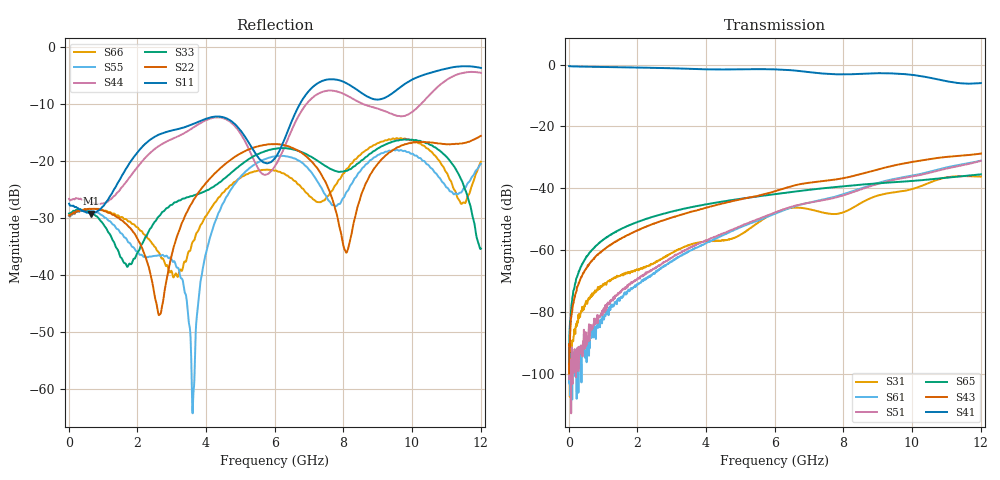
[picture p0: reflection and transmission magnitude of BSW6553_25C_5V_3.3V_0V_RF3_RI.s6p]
! Agilent Technologies	N5230C	MY49001333	A.09.33.09
!	Test time	=	2026-05-26
!	Product	=	BSW6553
!	Temp	=	25C
!	Logic	=	RF3
!	Port1	=	RFC
!	Port2	=	RF1
!	Port3	=	RF2
!	Port4	=	RF3
!	Port5	=	RF4
!	Port6	=	RF5
!S6P File: Measurements: <S11,S12,S13,S14,S15,S16>,
!<S21,S22,S23,S24,S25,S26>,
!<S31,S32,S33,S34,S35,S36>,
!<S41,S42,S43,S44,S45,S46>,
!<S51,S52,S53,S54,S55,S56>,
!<S61,S62,S63,S64,S65,S66>;
# HZ S RI R 50
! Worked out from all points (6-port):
!   1201 points, 10 MHz to 12.01 GHz, reference 50 ohm
!   strongest paths, dB at 10 MHz, 3.01 GHz, 6.01 GHz, 9.01 GHz, 12.01 GHz:
!     S41: -0.5, -1.2, -1.5, -2.8, -6.0
!     S43: -100.0, -49.5, -41.0, -34.0, -28.8
!     S65: -96.2, -47.6, -41.9, -38.4, -35.5
!     S51: -101.9, -62.4, -47.9, -38.6, -31.2
!     S61: -101.7, -63.7, -48.3, -38.3, -31.1
!     S31: -99.4, -60.9, -47.9, -42.4, -36.3
!   lowest |S11| = -29.2 dB at 650 MHz (marker M1), VSWR 1.07, Z = 49.2 - j3.33 ohm
!   |S11| at or under -10 dB: start of sweep to 6.732 GHz
